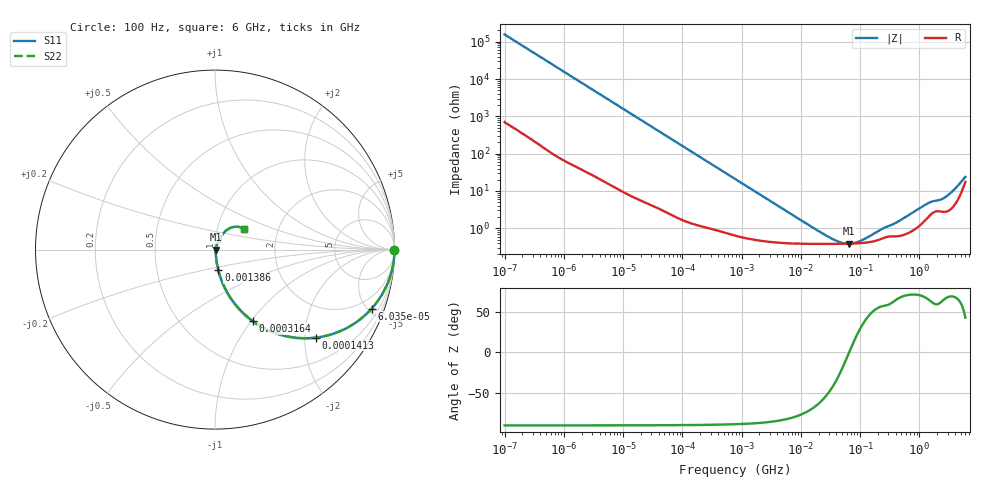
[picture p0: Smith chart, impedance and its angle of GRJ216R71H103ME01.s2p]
!Murata Part Number: GRJ216R71H103ME01
!These Parameters are Measured in Series Mode Connection
!Data Generated on Jun 19, 2026
!  o--ll--o
!Port1  Port2
!  o------o
!Operation Temp=25[degC], DC Bias Voltage=0[V]
!Freq. Start=100[Hz] Stop=6[GHz] 401[Steps]
# Hz S RI R 50
!Freq.(Hz) S11(Real) S11(Imag) S21(Real) S21(Imag) S12(Real) S12(Imag) S22(Real) S22(Imag)
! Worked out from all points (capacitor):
!   401 points, 100 Hz to 6 GHz, reference 50 ohm
!   read as one part in series: C = 10.2 nF near 109 Hz
!   lowest |Z| = 388 mohm at 65.19 MHz (marker M1)
!   series resonance near 65.52 MHz, so ESL is about 580 pH
!   S11 on the Smith chart (normalised r, x): 100 Hz: open; 60.35 kHz: 1.05, -5.28; 141.3 kHz: 1.03, -2.26; 316.4 kHz: 1.02, -1.02; 1.386 MHz: 1.01, -0.23; 6 GHz: 1.35, +0.32
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100  1 -0.000641  3.3e-06 0.000641  3.3e-06 0.000641  1 -0.000641
2008  0.9998 -0.0128  0.000224 0.0128  0.000224 0.0128  0.9998 -0.0128
12041  0.9938 -0.0756  0.00622 0.0756  0.00622 0.0756  0.9938 -0.0756
40335  0.9377 -0.2374  0.0623 0.2374  0.0623 0.2374  0.9377 -0.2374
60352  0.8722 -0.3293  0.1278 0.3293  0.1278 0.3293  0.8722 -0.3293
90302  0.7553 -0.4249  0.2447 0.4249  0.2447 0.4249  0.7553 -0.4249
141303  0.5607 -0.4904  0.4393 0.4904  0.4393 0.4904  0.5607 -0.4904
202169  0.3872 -0.4799  0.6128 0.4799  0.6128 0.4799  0.3872 -0.4799
316350  0.2094 -0.3976  0.7906 0.3976  0.7906 0.3976  0.2094 -0.3976
473344  0.1096 -0.3009  0.8904 0.3009  0.8904 0.3009  0.1096 -0.3009
774597  0.0475 -0.1979  0.9525 0.1979  0.9525 0.1979  0.0475 -0.1979
1386327  0.0185 -0.1146  0.9815 0.1146  0.9815 0.1146  0.0185 -0.1146
3712478  0.00608 -0.0436  0.9939 0.0436  0.9939 0.0436  0.00608 -0.0436
1.555665e7  0.00391 -0.00992  0.9961 0.00992  0.9961 0.00992  0.00391 -0.00992
3.80911e7  0.00382 -0.00284  0.9962 0.00284  0.9962 0.00284  0.00382 -0.00284
6.518806e7  0.00386 -2.5e-05  0.9961 2.5e-05  0.9961 2.5e-05  0.00386 -2.5e-05
1.066761e8  0.00402 0.00253  0.996 -0.00253  0.996 -0.00253  0.00402 0.00253
3.124326e8  0.00609 0.00991  0.9939 -0.00991  0.9939 -0.00991  0.00609 0.00991
1.369159e9  0.0202 0.0403  0.9798 -0.0403  0.9798 -0.0403  0.0202 0.0403
2.562649e9  0.0298 0.0541  0.9702 -0.0541  0.9702 -0.0541  0.0298 0.0541
4.193612e9  0.0573 0.1022  0.9427 -0.1022  0.9427 -0.1022  0.0573 0.1022
6e9  0.1643 0.114  0.8357 -0.114  0.8357 -0.114  0.1643 0.114
